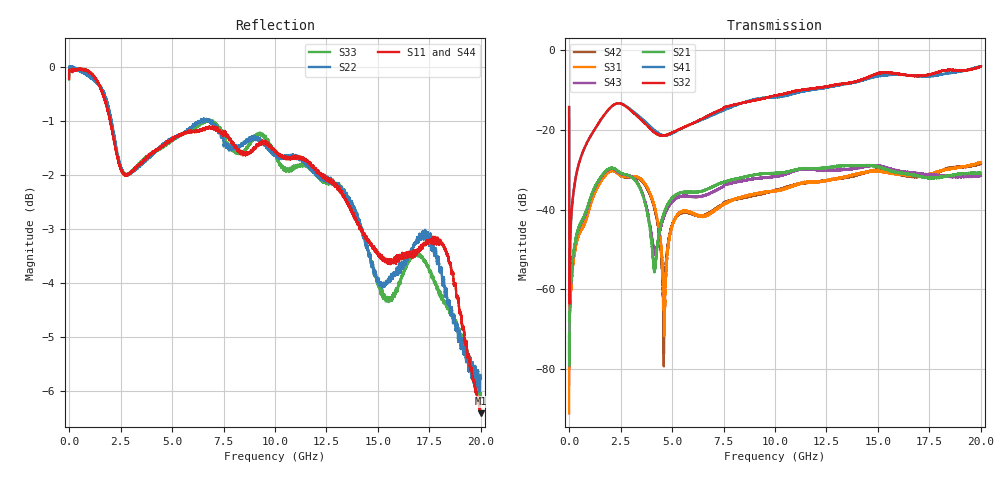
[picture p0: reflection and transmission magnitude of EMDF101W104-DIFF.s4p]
!EMDF101W104
!Johanson Technology Inc.
!www.johansontechnology.com
!Test Board Conditions:
!Substrate Type  RO4350B
!Substrate Thickness  21 mil
!Substrate Dk  3.66
!TL Type: GCPW
!TL Trace Width  40 mil
!TL Gap  17.5 mil
!PART MODE DIFFERENTIAL
!DUT TOPOLOGY	DIFFERENTIAL 4-PORT
# MHz S  dB  R 50
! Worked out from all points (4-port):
!   20001 points, 300 kHz to 20 GHz, reference 50 ohm
!   strongest paths, dB at 300 kHz, 5 GHz, 10 GHz, 15 GHz, 20 GHz:
!     S32: -14.2, -20.6, -11.4, -5.8, -4.0
!     S41: -14.2, -20.9, -11.8, -6.5, -4.0
!     S21: -71.5, -37.1, -30.8, -29.2, -30.8
!     S43: -71.8, -38.0, -31.7, -29.0, -31.5
!     S31: -91.2, -44.2, -35.3, -30.4, -28.1
!     S42: -73.6, -43.8, -35.2, -30.0, -28.4
!   lowest |S11| = -6.4 dB at 20 GHz (marker M1), VSWR 2.83, Z = 22.5 - j24 ohm
!   |S11| at or under -10 dB: nowhere
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0.3  -0.21 -168.8  -71.27 -71.5  -75.24 -122.0  -14.18 -78.1
     -71.54 -37.2  -0.16 -168.8  -14.26 -78.4  -71.84 -30.9
     -91.22 48.9  -14.22 -78.1  -0.23 -168.9  -88.35 -176.1
     -14.22 -78.1  -73.64 -103.8  -71.85 -81.4  -0.09 -168.7
374.294  -0.05 174.3  -46.08 74.8  -47.88 72.8  -30.45 77.9
         -46.08 74.0  -0.03 174.1  -30.58 78.5  -48.10 72.3
         -47.89 71.9  -30.57 78.2  -0.04 174.8  -46.46 74.3
         -30.54 78.3  -48.09 72.5  -46.34 74.4  0.00 174.1
1967.27  -0.95 145.4  -29.53 17.8  -30.47 13.8  -14.56 33.8
         -29.62 17.9  -0.82 146.3  -14.60 34.6  -30.46 14.1
         -30.45 13.8  -14.53 34.5  -0.90 149.3  -29.75 21.0
         -14.61 33.9  -30.46 13.8  -29.82 21.0  -0.86 149.3
4604.231  -1.44 123.3  -40.96 27.6  -64.73 -128.4  -21.32 -25.6
          -40.90 27.4  -1.43 121.8  -21.39 -19.1  -69.03 -36.8
          -64.89 -127.4  -21.39 -19.3  -1.47 128.2  -41.72 18.3
          -21.32 -25.2  -70.32 -9.0  -41.73 19.9  -1.40 127.1
11784.12  -1.84 14.4  -29.63 -100.5  -33.03 -124.8  -9.98 -81.5
          -29.67 -101.0  -1.89 19.0  -9.53 -78.8  -33.12 -121.8
          -33.05 -124.7  -9.57 -78.0  -1.91 29.9  -29.88 -90.2
          -9.92 -82.3  -33.13 -121.2  -29.79 -91.0  -1.97 29.5
19997  -6.41 -120.5  -30.91 62.9  -28.12 48.9  -4.25 147.0
       -30.83 63.1  -5.75 -113.1  -3.79 151.8  -28.55 52.6
       -28.08 48.7  -4.00 152.3  -6.09 -91.6  -31.67 92.4
       -3.97 146.2  -28.41 52.1  -31.39 91.4  -6.22 -89.6
20000  -6.40 -120.6  -30.98 63.1  -28.16 48.9  -4.25 146.9
       -30.82 62.3  -5.77 -113.0  -3.83 151.8  -28.51 52.5
       -28.10 48.7  -4.01 152.2  -6.09 -91.6  -31.64 92.0
       -3.97 146.1  -28.42 51.9  -31.50 91.5  -6.23 -89.6
